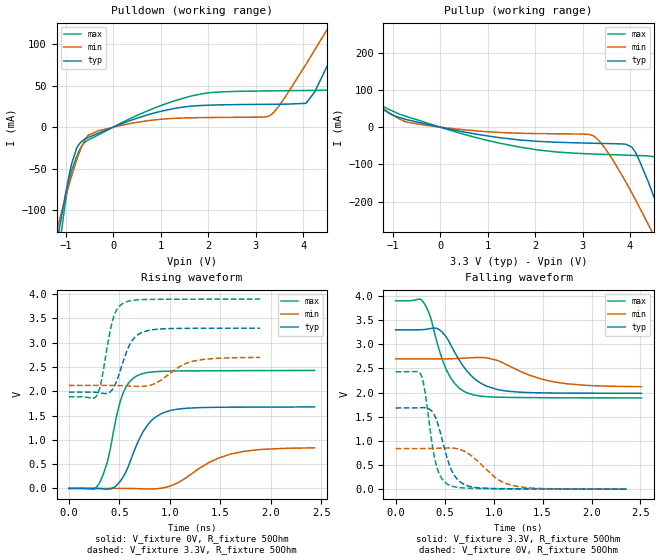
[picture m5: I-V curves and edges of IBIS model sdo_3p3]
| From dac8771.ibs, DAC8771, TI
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|   sdo_3p3 Model
[Model]   sdo_3p3
Model_type   Output
Polarity   Non-Inverting
Vmeas = 1.65
Vref = 0
Cref = 2pF
Rref = 140
|   typ   min   max
|   (nom PVT)   (fast PVT)   (slow PVT)
C_comp   2.914e-12   2.914e-12   3.015e-12
| Where nom  PVT is Nominal Process, 3.3V, 27C
|   Fast PVT is Strong Process,  3.9V, -40C
|   Slow PVT is Weak Process,   2.7V, 150C
[Voltage Range]   3.3   2.7   3.9
|Junction Temperature
[Temperature Range]   27   150   -40
[Pullup Reference]   3.3   2.7   3.9
[Pulldown Reference]   0   0   0
[Power Clamp Reference]   3.3   2.7   3.9
[GND Clamp Reference]   0   0   0
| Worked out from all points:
|   slope of the pulldown table from 0 to 0.495 V, typ, clamps not added: 46.7 ohm
|   slope of the pullup table from 0 to 0.495 V, typ, clamps not added: 38.8 ohm
|   falling waveform, V_fixture 3.3V, R_fixture 50Ohm: 20-80 % time 281ps typ, 452ps min, 202ps max; typ from 3.3 V to 1.99 V
|   rising waveform, V_fixture 0V, R_fixture 50Ohm: 20-80 % time 231ps typ, 424ps min, 162ps max; typ from 0 V to 1.68 V
|   rising waveform, V_fixture 3.3V, R_fixture 50Ohm: 20-80 % time 144ps typ, 255ps min, 109ps max; typ from 1.98 V to 3.3 V
|   falling waveform, V_fixture 0V, R_fixture 50Ohm: 20-80 % time 153ps typ, 288ps min, 111ps max; typ from 1.68 V to 0.005 V
[Pulldown]
|   Voltage   I(typ)   I(min)   I(max)
-3.3V     -923.4mA   -672.4mA   -1.168A
-1.201V   -141.9mA   -125.7mA   -170.5mA
-1.026V   -85.06mA   -87.71mA   -95.4mA
-772.2mV  -24.7mA    -39.05mA   -34.87mA
-535.2mV  -12.47mA   -10.01mA   -15.58mA
1.466V    24.12mA    10.98mA    34.68mA
3.231V    27.44mA    12.44mA    43.57mA
4.059V    28.6mA     75.5mA     44.04mA
4.676V    93.54mA    133.5mA    44.58mA
4.844V    114.6mA    149.6mA    51.83mA
5.331V    176.2mA    196.2mA    125.6mA
6.6V      340mA      319mA      337.8mA
[Pullup]
|   Voltage   I(typ)   I(min)   I(max)
-3.3V     310mA      247.8mA    391.3mA
-1.841V   124.2mA    108.6mA    148.5mA
-996.9mV  32.03mA    32.08mA    42.58mA
1.251V    -28.29mA   -14.33mA   -43.09mA
3.151V    -43.04mA   -19.87mA   -71.72mA
3.92V     -46.14mA   -149.3mA   -75.23mA
4.122V    -69.45mA   -196.6mA   -76.06mA
4.375V    -143.9mA   -258.6mA   -77.13mA
4.753V    -275mA     -355.5mA   -108mA
5.115V    -407.7mA   -451.3mA   -253.6mA
5.257V    -460.5mA   -489.5mA   -319.5mA
6.6V      -970.6mA   -861.8mA   -962.9mA
[Ramp]
R_load = 50
|   typ   min   max
dV/dt_r   1.00955/2.31715e-10   0.506532/4.27537e-10   1.45927/1.62663e-10
dV/dt_f   0.790767/2.82458e-10   0.348658/4.61019e-10   1.20872/2.0231e-10
[Falling Waveform]
V_fixture = 3.3V
V_fixture_min = 2.7V
V_fixture_max = 3.9V
R_fixture = 50Ohm
|   Time   V(typ)   V(min)   V(max)
0s        3.3V       2.7V       3.9V
282.8ps   3.304V     2.7V       3.873V
354.3ps   3.326V     2.699V     3.567V
417.4ps   3.331V     2.699V     3.076V
530ps     3.111V     2.7V       2.423V
739.8ps   2.419V     2.719V     1.988V
907.2ps   2.155V     2.724V     1.921V
1.142ns   2.032V     2.569V     1.902V
1.647ns   1.992V     2.213V     1.895V
2.51ns    1.987V     2.125V     1.89V
[Rising Waveform]
V_fixture = 0V
V_fixture_min = 0V
V_fixture_max = 0V
R_fixture = 50Ohm
|   Time   V(typ)   V(min)   V(max)
0s        2.122nV    12.53nV    2.171nV
298.3ps   -3.131mV   317.2uV    93.77mV
384ps     -15.45mV   665.5uV    566.7mV
471.8ps   60.67mV    771.7uV    1.477V
530ps     208.8mV    342.2uV    1.915V
676.7ps   917.6mV    -4.753mV   2.319V
818.2ps   1.394V     -12.5mV    2.395V
1.034ns   1.616V     73.47mV    2.415V
1.618ns   1.672V     713.8mV    2.423V
2.435ns   1.676V     834.4mV    2.427V
[Rising Waveform]
V_fixture = 3.3V
V_fixture_min = 2.7V
V_fixture_max = 3.9V
R_fixture = 50Ohm
|   Time   V(typ)   V(min)   V(max)
0s        1.982V     2.119V     1.885V
241.1ps   1.981V     2.119V     1.857V
286.1ps   1.973V     2.12V      1.948V
325.3ps   1.96V      2.12V      2.238V
439.9ps   2.062V     2.119V     3.506V
545.7ps   2.656V     2.114V     3.82V
640.7ps   3.08V      2.103V     3.873V
777ps     3.245V     2.109V     3.889V
1.221ns   3.295V     2.614V     3.895V
1.895ns   3.297V     2.696V     3.897V
[Falling Waveform]
V_fixture = 0V
V_fixture_min = 0V
V_fixture_max = 0V
R_fixture = 50Ohm
|   Time   V(typ)   V(min)   V(max)
0s        1.683V     844.2mV    2.432V
262.1ps   1.69V      843.5mV    2.353V
301.9ps   1.687V     844.2mV    1.987V
408.8ps   1.474V     848.6mV    544.9mV
536.1ps   575mV      856.3mV    99.06mV
598.3ps   290.8mV    850.1mV    53.49mV
703ps     97.65mV    786.7mV    28.09mV
1.044ns   13.67mV    205.3mV    15.25mV
1.227ns   10.28mV    64.82mV    13.03mV
2.362ns   5.295mV    4.058mV    5.775mV
